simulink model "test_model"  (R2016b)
settings: Solver=VariableStepAuto  StartTime=0.0  StopTime=runtime  RelTol=1e-3
InitFcn:
  | clear mex
  | delete test_model_sfun.mexw64
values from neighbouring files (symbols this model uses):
  g = 9.81    [modelParameters.m]
  height_controlled_o = (((Rm*If        + (((omega0_o * 2 * Rm * Kv * Kq      * Kd + 1)^2) - 1)/(4* Rm*Kv^2*Kq      * Kd))/Vb)*(Pmax - Pmin) + Pmin)    [modelParameters.m]
  If = 0.3836    [modelParameters.m]
  Jreq = 4.2012e-05    [modelParameters.m]
  Jxx = 0.0130    (= 0.013)    [modelParameters.m]
  Jyy = 0.0140    (= 0.014)    [modelParameters.m]
  Jzz = 0.0285    [modelParameters.m]
  Kd = 1.4852e-07    [modelParameters.m]
  Ki_mahony = 0.001    [modelParameters.m]
  Kp_mahony = 0.4    [modelParameters.m]
  Kq = 96.3422    [modelParameters.m]
  Kt = 1.2007e-05    [modelParameters.m]
  Kv = 96.3422    [modelParameters.m]
  m = 1.216    [modelParameters.m]
  omega0_o = sqrt((m*g)/(4*Kt))    [modelParameters.m]
  omega1_o = sqrt((m*g)/(4*Kt))    [modelParameters.m]
  omega2_o = sqrt((m*g)/(4*Kt))    [modelParameters.m]
  omega3_o = sqrt((m*g)/(4*Kt))    [modelParameters.m]
  pitch_o = 0    [modelParameters.m]
  pitchrate_o = 0    [modelParameters.m]
  Pmax = 1    [modelParameters.m]
  Pmin = 0    [modelParameters.m]
  r_oc = [0; 0; 0]    [modelParameters.m]
  rhx = 0.16    [modelParameters.m]
  rhy = 0.16    [modelParameters.m]
  rhz = 0.03    [modelParameters.m]
  Rm = 0.235    [modelParameters.m]
  roll_o = 0    [modelParameters.m]
  rollrate_o = 0    [modelParameters.m]
  Tc = 0.04    [modelParameters.m]
  Tq = 0.005    [modelParameters.m]
  Vb = 11.4    [modelParameters.m]
  x_controlled_o = 0    [modelParameters.m]
  x_o = 0    [modelParameters.m]
  x_vel_o = 0    [modelParameters.m]
  y_controlled_o = 0    [modelParameters.m]
  y_o = 0    [modelParameters.m]
  y_vel_o = 0    [modelParameters.m]
  yaw_controlled_o = 0    [modelParameters.m]
  yaw_o = 0    [modelParameters.m]
  yawrate_o = 0    [modelParameters.m]
  z_o = 0    [modelParameters.m]
  z_vel_o = 0    [modelParameters.m]
undefined symbols (not defined in the file or in its folder): a, Ki, Kp, Ts
libraries: simulink x38, dsparch4 x3, vrlib x2
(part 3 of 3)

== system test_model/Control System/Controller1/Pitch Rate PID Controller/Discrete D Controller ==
  pitch_angle : Inport
  Discrete Derivative : simulink/Discrete/Discrete Derivative  gainval=Kd  ICPrevScaledInput=0.0  OutMin=[]  OutMax=[]  OutDataType=fixdt(1, 16)  OutScaling=2^-10  DoSatur=off
  Discrete Filter : DiscreteFilter  Numerator=[0 a]  Denominator=[1-a]
  Sum : Sum  Inputs=|++
  output : Outport
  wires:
  Discrete Derivative/1 -> Sum/1
  Discrete Filter/1 -> Sum/2
  Sum/1 -> Discrete Filter/1, output/1
  pitch_angle/1 -> Discrete Derivative/1

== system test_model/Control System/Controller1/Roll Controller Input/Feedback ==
  roll_error_model : Inport
  roll_error : Outport
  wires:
  roll_error_model/1 -> roll_error/1

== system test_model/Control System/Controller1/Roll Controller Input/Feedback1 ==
  roll_angle_model : Inport
  roll_angle : Outport
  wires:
  roll_angle_model/1 -> roll_angle/1

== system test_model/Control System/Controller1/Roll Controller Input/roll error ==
  From Workspace1 : FromWorkspace  VariableName=roll_angle  SampleTime=Tq  Interpolate=off  OutputAfterFinalValue=Holding final value
  From Workspace4 : FromWorkspace  VariableName=roll_error  SampleTime=Tq  Interpolate=off  OutputAfterFinalValue=Holding final value
  roll_error : Outport
  roll_angle : Outport  Port=2
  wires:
  From Workspace4/1 -> roll_error/1
  From Workspace1/1 -> roll_angle/1

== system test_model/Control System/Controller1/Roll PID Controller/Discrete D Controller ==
  pitch_angle : Inport
  Discrete Derivative : simulink/Discrete/Discrete Derivative  gainval=Kd  ICPrevScaledInput=0.0  OutMin=[]  OutMax=[]  OutDataType=fixdt(1, 16)  OutScaling=2^-10  DoSatur=off
  Discrete Filter : DiscreteFilter  Numerator=[0 a]  Denominator=[1-a]
  Sum : Sum  Inputs=|++
  output : Outport
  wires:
  Discrete Derivative/1 -> Sum/1
  Discrete Filter/1 -> Sum/2
  Sum/1 -> Discrete Filter/1, output/1
  pitch_angle/1 -> Discrete Derivative/1

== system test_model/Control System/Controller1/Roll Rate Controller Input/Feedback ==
  rollrate_error_model : Inport
  rollrate_error : Outport
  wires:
  rollrate_error_model/1 -> rollrate_error/1

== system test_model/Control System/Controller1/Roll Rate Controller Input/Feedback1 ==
  rollrate_model : Inport
  rollrate : Outport
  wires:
  rollrate_model/1 -> rollrate/1

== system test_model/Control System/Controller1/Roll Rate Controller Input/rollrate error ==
  From Workspace1 : FromWorkspace  VariableName=rollrate  SampleTime=Tq  Interpolate=off  OutputAfterFinalValue=Holding final value
  From Workspace5 : FromWorkspace  VariableName=rollrate_error  SampleTime=Tq  Interpolate=off  OutputAfterFinalValue=Holding final value
  rollrate_error : Outport
  rollrate : Outport  Port=2
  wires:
  From Workspace5/1 -> rollrate_error/1
  From Workspace1/1 -> rollrate/1

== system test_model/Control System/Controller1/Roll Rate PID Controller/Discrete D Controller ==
  pitch_angle : Inport
  Discrete Derivative : simulink/Discrete/Discrete Derivative  gainval=Kd  ICPrevScaledInput=0.0  OutMin=[]  OutMax=[]  OutDataType=fixdt(1, 16)  OutScaling=2^-10  DoSatur=off
  Discrete Filter : DiscreteFilter  Numerator=[0 a]  Denominator=[1-a]
  Sum : Sum  Inputs=|++
  output : Outport
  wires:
  Discrete Derivative/1 -> Sum/1
  Discrete Filter/1 -> Sum/2
  Sum/1 -> Discrete Filter/1, output/1
  pitch_angle/1 -> Discrete Derivative/1

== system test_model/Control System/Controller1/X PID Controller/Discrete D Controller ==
  x_pos : Inport
  Discrete Derivative : simulink/Discrete/Discrete Derivative  gainval=Kd  ICPrevScaledInput=0.0  OutMin=[]  OutMax=[]  OutDataType=fixdt(1, 16)  OutScaling=2^-10  DoSatur=off
  Discrete Filter : DiscreteFilter  Numerator=[0 a]  Denominator=[1-a]
  Sum : Sum  Inputs=|++
  output : Outport
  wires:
  Discrete Derivative/1 -> Sum/1
  Discrete Filter/1 -> Sum/2
  Sum/1 -> Discrete Filter/1, output/1
  x_pos/1 -> Discrete Derivative/1

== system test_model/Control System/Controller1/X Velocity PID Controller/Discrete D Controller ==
  x_vel : Inport
  Discrete Derivative : simulink/Discrete/Discrete Derivative  gainval=1.0  ICPrevScaledInput=0.0  OutMin=[]  OutMax=[]  OutDataType=fixdt(1, 16)  OutScaling=2^-10  DoSatur=off
  Discrete Filter : DiscreteFilter  Numerator=[0 a]  Denominator=[1-a]
  Sum : Sum  Inputs=|++
  output : Outport
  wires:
  Discrete Derivative/1 -> Sum/1
  Discrete Filter/1 -> Sum/2
  Sum/1 -> Discrete Filter/1, output/1
  x_vel/1 -> Discrete Derivative/1

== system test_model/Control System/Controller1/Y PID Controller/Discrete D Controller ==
  y_pos : Inport
  Discrete Derivative : simulink/Discrete/Discrete Derivative  gainval=1.0  ICPrevScaledInput=0.0  OutMin=[]  OutMax=[]  OutDataType=fixdt(1, 16)  OutScaling=2^-10  DoSatur=off
  Discrete Filter : DiscreteFilter  Numerator=[0 a]  Denominator=[1-a]
  Sum : Sum  Inputs=|++
  output : Outport
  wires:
  Discrete Derivative/1 -> Sum/1
  Discrete Filter/1 -> Sum/2
  Sum/1 -> Discrete Filter/1, output/1
  y_pos/1 -> Discrete Derivative/1

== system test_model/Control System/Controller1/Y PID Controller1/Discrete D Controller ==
  y_pos : Inport
  Discrete Derivative : simulink/Discrete/Discrete Derivative  gainval=1.0  ICPrevScaledInput=0.0  OutMin=[]  OutMax=[]  OutDataType=fixdt(1, 16)  OutScaling=2^-10  DoSatur=off
  Discrete Filter : DiscreteFilter  Numerator=[0 a]  Denominator=[1-a]
  Sum : Sum  Inputs=|++
  output : Outport
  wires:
  Discrete Derivative/1 -> Sum/1
  Discrete Filter/1 -> Sum/2
  Sum/1 -> Discrete Filter/1, output/1
  y_pos/1 -> Discrete Derivative/1

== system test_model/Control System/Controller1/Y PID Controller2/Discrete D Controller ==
  x_pos : Inport
  Discrete Derivative : simulink/Discrete/Discrete Derivative  gainval=1.0  ICPrevScaledInput=0.0  OutMin=[]  OutMax=[]  OutDataType=fixdt(1, 16)  OutScaling=2^-10  DoSatur=off
  Discrete Filter : DiscreteFilter  Numerator=[0 a]  Denominator=[1-a]
  Sum : Sum  Inputs=|++
  output : Outport
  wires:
  Discrete Derivative/1 -> Sum/1
  Discrete Filter/1 -> Sum/2
  Sum/1 -> Discrete Filter/1, output/1
  x_pos/1 -> Discrete Derivative/1

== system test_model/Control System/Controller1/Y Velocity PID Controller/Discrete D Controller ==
  y_pos : Inport
  Discrete Derivative : simulink/Discrete/Discrete Derivative  gainval=1.0  ICPrevScaledInput=0.0  OutMin=[]  OutMax=[]  OutDataType=fixdt(1, 16)  OutScaling=2^-10  DoSatur=off
  Discrete Filter : DiscreteFilter  Numerator=[0 a]  Denominator=[1-a]
  Sum : Sum  Inputs=|++
  output : Outport
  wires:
  Discrete Derivative/1 -> Sum/1
  Discrete Filter/1 -> Sum/2
  Sum/1 -> Discrete Filter/1, output/1
  y_pos/1 -> Discrete Derivative/1

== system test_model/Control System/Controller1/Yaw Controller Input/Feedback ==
  yaw_error_model : Inport
  yaw_error : Outport
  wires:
  yaw_error_model/1 -> yaw_error/1

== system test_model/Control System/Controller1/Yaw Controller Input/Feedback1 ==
  yaw_angle_model : Inport
  yaw_angle : Outport
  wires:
  yaw_angle_model/1 -> yaw_angle/1

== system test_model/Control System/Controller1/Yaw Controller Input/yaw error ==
  From Workspace1 : FromWorkspace  VariableName=yaw_angle  SampleTime=Tc  Interpolate=off  OutputAfterFinalValue=Holding final value
  From Workspace7 : FromWorkspace  VariableName=yaw_error  SampleTime=Tc  Interpolate=off  OutputAfterFinalValue=Holding final value
  yaw_error : Outport
  yaw_angle : Outport  Port=2
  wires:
  From Workspace7/1 -> yaw_error/1
  From Workspace1/1 -> yaw_angle/1

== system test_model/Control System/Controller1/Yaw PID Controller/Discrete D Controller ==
  yaw_pos : Inport
  Discrete Derivative : simulink/Discrete/Discrete Derivative  gainval=1.0  ICPrevScaledInput=0.0  OutMin=[]  OutMax=[]  OutDataType=fixdt(1, 16)  OutScaling=2^-10  DoSatur=off
  Discrete Filter : DiscreteFilter  Numerator=[0 a]  Denominator=[1-a]
  Sum : Sum  Inputs=|++
  output : Outport
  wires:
  Discrete Derivative/1 -> Sum/1
  Discrete Filter/1 -> Sum/2
  Sum/1 -> Discrete Filter/1, output/1
  yaw_pos/1 -> Discrete Derivative/1

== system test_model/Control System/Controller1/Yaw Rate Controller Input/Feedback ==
  yawrate_error_model : Inport
  yawrate_error : Outport
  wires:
  yawrate_error_model/1 -> yawrate_error/1

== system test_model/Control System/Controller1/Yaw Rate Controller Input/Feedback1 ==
  yawrate_model : Inport
  yawrate : Outport
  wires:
  yawrate_model/1 -> yawrate/1

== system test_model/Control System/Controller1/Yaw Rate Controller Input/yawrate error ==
  From Workspace1 : FromWorkspace  VariableName=yawrate  SampleTime=Tq  Interpolate=off  OutputAfterFinalValue=Holding final value
  From Workspace8 : FromWorkspace  VariableName=yawrate_error  SampleTime=Tq  Interpolate=off  OutputAfterFinalValue=Holding final value
  yawrate_error : Outport
  yawrate : Outport  Port=2
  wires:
  From Workspace8/1 -> yawrate_error/1
  From Workspace1/1 -> yawrate/1

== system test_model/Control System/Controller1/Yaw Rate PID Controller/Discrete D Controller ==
  yawrate : Inport
  Discrete Derivative : simulink/Discrete/Discrete Derivative  gainval=Kd  ICPrevScaledInput=0.0  OutMin=[]  OutMax=[]  OutDataType=fixdt(1, 16)  OutScaling=2^-10  DoSatur=off
  Discrete Filter : DiscreteFilter  Numerator=[0 a]  Denominator=[1-a]
  Sum : Sum  Inputs=|++
  output : Outport
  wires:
  Discrete Derivative/1 -> Sum/1
  Discrete Filter/1 -> Sum/2
  Sum/1 -> Discrete Filter/1, output/1
  yawrate/1 -> Discrete Derivative/1

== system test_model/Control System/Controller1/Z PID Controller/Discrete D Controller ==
  z_pos : Inport
  Discrete Derivative : simulink/Discrete/Discrete Derivative  gainval=1.0  ICPrevScaledInput=0.0  OutMin=[]  OutMax=[]  OutDataType=fixdt(1, 16)  OutScaling=2^-10  DoSatur=off
  Discrete Filter : DiscreteFilter  Numerator=[0 a]  Denominator=[1-a]
  Sum : Sum  Inputs=|++
  output : Outport
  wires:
  Discrete Derivative/1 -> Sum/1
  Discrete Filter/1 -> Sum/2
  Sum/1 -> Discrete Filter/1, output/1
  z_pos/1 -> Discrete Derivative/1

== matlab function test_model/Actuation/Gravity

 ==
function E_Fg = gravity(m, g)

E_Fg = [0; 0; m*g];

== matlab function test_model/Actuation/Lbe





 ==
function E_ro  = linear_body_earth_conversion(B_vo, euler_angles)

euler_rates = zeros(3,1);
E_ro = zeros(3,1);

phi = euler_angles(1);
theta = euler_angles(2);
psi = euler_angles(3);

Leb = [cos(theta)*cos(psi), sin(phi)*sin(theta)*cos(psi)-cos(phi)*sin(psi), cos(phi)*sin(theta)*cos(psi)+sin(phi)*sin(psi); ...
       cos(theta)*sin(psi), sin(phi)*sin(theta)*sin(psi)+cos(phi)*cos(psi), cos(phi)*sin(theta)*sin(psi)-sin(phi)*cos(psi); ...
           -sin(theta)    ,                sin(phi)*cos(theta)            ,                 cos(phi)*cos(theta)           ];

E_ro = Leb * B_vo;

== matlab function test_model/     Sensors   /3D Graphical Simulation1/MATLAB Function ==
function y = eigenaxis_ucart(u)


if abs(u(1))< 0.0001
    u(1) = 0.0001;
end

if abs(u(2))< 0.0001
    u(2) = 0.0001;
end

if abs(u(3))< 0.0001
    u(3) = 0.0001;
end

u = [ -u(1); -u(2); u(3) ];% [Pitch, Yaw, Roll] 

C11 = cos(u(2))*cos(u(3));
C12 = cos(u(2))*sin(u(3));
C13 = -sin(u(2));
C21 = sin(u(1))*sin(u(2))*cos(u(3))-cos(u(1))*sin(u(3));
C22 = sin(u(1))*sin(u(2))*sin(u(3))+cos(u(1))*cos(u(3));
C23 = sin(u(1))*cos(u(2));
C31 = cos(u(1))*sin(u(2))*cos(u(3))+sin(u(1))*sin(u(3));
C32 = cos(u(1))*sin(u(2))*sin(u(3))-sin(u(1))*cos(u(3));
C33 = cos(u(1))*cos(u(2));
    
theta = acos(0.5*(C11+C22+C33-1));

e = [C23-C32; C31-C13; C12-C21]/(2*sin(theta));
    
y = [e; theta];

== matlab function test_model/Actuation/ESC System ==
function Vb_eff   = ESC(P, Pmin, Pmax, Vb)

P1 = P(1);
P2 = P(2);
P3 = P(3);
P4 = P(4);

% Define u_Pi for each of the rotors, limiting it to be greater than 0
% u_P0 = (rotor_0_duty_cycle/100 - Pmin) / (Pmax - Pmin);
% u_P1 = (rotor_1_duty_cycle/100 - Pmin) / (Pmax - Pmin);
% u_P2 = (rotor_2_duty_cycle/100 - Pmin) / (Pmax - Pmin);
% u_P3 = (rotor_3_duty_cycle/100 - Pmin) / (Pmax - Pmin);
u_P0 = (P1 - Pmin) / (Pmax - Pmin);
u_P1 = (P2 - Pmin) / (Pmax - Pmin);
u_P2 = (P3 - Pmin) / (Pmax - Pmin);
u_P3 = (P4 - Pmin) / (Pmax - Pmin);


% Determine the effective battery voltage from each ESC
Vb_eff_0 = u_P0 * Vb;
Vb_eff_1 = u_P1 * Vb;
Vb_eff_2 = u_P2 * Vb;
Vb_eff_3 = u_P3 * Vb;
    
Vb_eff = [Vb_eff_0, Vb_eff_1, Vb_eff_2, Vb_eff_3];

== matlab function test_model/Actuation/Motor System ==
function w_dot = motor(Vb_eff, w, Rm, Kv, Kq, Kd, If, Jreq)

% Define each motors effective battery voltage
Vb_eff_0 = Vb_eff(1);
Vb_eff_1 = Vb_eff(2);
Vb_eff_2 = Vb_eff(3);
Vb_eff_3 = Vb_eff(4);

% Determine the angular velocity of each rotor from feedback
w_0 = w(1);
w_1 = w(2);
w_2 = w(3);
w_3 = w(4);

% Determine angular acceleration of each rotor
w_0_dot = 1/(Jreq*Rm*Kq) * Vb_eff_0 - 1/(Jreq*Rm*Kq*Kv) * w_0 - 1/(Jreq*Kq)*If - (Kd/Jreq) * w_0^2;
w_1_dot = 1/(Jreq*Rm*Kq) * Vb_eff_1 - 1/(Jreq*Rm*Kq*Kv) * w_1 - 1/(Jreq*Kq)*If - (Kd/Jreq) * w_1^2;
w_2_dot = 1/(Jreq*Rm*Kq) * Vb_eff_2 - 1/(Jreq*Rm*Kq*Kv) * w_2 - 1/(Jreq*Kq)*If - (Kd/Jreq) * w_2^2;
w_3_dot = 1/(Jreq*Rm*Kq) * Vb_eff_3 - 1/(Jreq*Rm*Kq*Kv) * w_3 - 1/(Jreq*Kq)*If - (Kd/Jreq) * w_3^2;

w_dot = [w_0_dot, w_1_dot, w_2_dot, w_3_dot];

== matlab function test_model/Actuation/Rotor System







 ==
function [B_omega_dot, B_vo_dot]= rotor(w_dot, w, B_Fg, B_omega, B_vo, m, Kt, Kd, rhx, rhy, rhz, Jreq, Jxx, Jyy, Jzz, r_oc)

% Create J vector
J = [Jxx,  0 ,  0 ; ...
      0 , Jyy,  0 ; ...
      0 ,  0 , Jzz;];
  
r_oc_X = [0, -r_oc(3), r_oc(2); r_oc(3), 0, -r_oc(1); -r_oc(2), r_oc(1), 0];

% Create r_hi vector
rh_0 = [-rhx; rhy; -rhz];
rh_1 = [rhx; rhy; -rhz];
rh_2 = [-rhx; -rhy; -rhz];
rh_3 = [rhx; -rhy; -rhz];

% Define 3x3 Identity Matrix
I = eye(3);

% Create gamma vectors
gamma_Ti = [0; 0; -1];
gamma_omega_03 = [0; 0; 1];  %Rotors 0 and 3 use this gamma_omega vector
gamma_omega_12 = [0; 0; -1]; %Rotors 1 and 2 use this gamma_omega vector

% Define angular velocities for each rotor
w_0 = w(1);
w_1 = w(2);
w_2 = w(3);
w_3 = w(4);

% Define angular acceleration for each rotor
w_0_dot = w_dot(1);
w_1_dot = w_dot(2);
w_2_dot = w_dot(3);
w_3_dot = w_dot(4);

% Define the rotor force in the z-direction from each rotor
B_Fr_0 = Kt * w_0 * w_0 * gamma_Ti;
B_Fr_1 = Kt * w_1 * w_1 * gamma_Ti;
B_Fr_2 = Kt * w_2 * w_2 * gamma_Ti;
B_Fr_3 = Kt * w_3 * w_3 * gamma_Ti;

% Sum up the rotor forces in the z-direction from each vector to get the
% total body force in the z-direction
B_Fr = B_Fr_0 + B_Fr_1 + B_Fr_2 + B_Fr_3;

% Define the in-plane drag and induced torque produced by each rotor
 B_Q_d0 = -1 * Kd * w_0 * w_0 * gamma_omega_03;
 B_Q_d1 = -1 * Kd * w_1 * w_1 * gamma_omega_12;
 B_Q_d2 = -1 * Kd * w_2 * w_2 * gamma_omega_12;
 B_Q_d3 = -1 * Kd * w_3 * w_3 * gamma_omega_03;

% Sum up the total in-plane drag and induced torque to get the total
% in-plane drag and induced torque on the body
B_Q_d = B_Q_d0 + B_Q_d1 + B_Q_d2 + B_Q_d3;

% Define the force lever arm torque created from the force produced by each
% rotor in the z-direction
B_Q_F0 = cross( rh_0, B_Fr_0 );
B_Q_F1 = cross( rh_1, B_Fr_1 );
B_Q_F2 = cross( rh_2, B_Fr_2 );
B_Q_F3 = cross( rh_3, B_Fr_3 );

B_Q_F = B_Q_F0 + B_Q_F1 + B_Q_F2 + B_Q_F3;

%Define the change in angular momentum torque produced by each rotor 
B_Q_L0 = -1 * Jreq * ( cross(B_omega, w_0 * gamma_omega_03) + w_0_dot * gamma_omega_03 );
B_Q_L1 = -1 * Jreq * ( cross(B_omega, w_1 * gamma_omega_12) + w_1_dot * gamma_omega_12 ); 
B_Q_L2 = -1 * Jreq * ( cross(B_omega, w_2 * gamma_omega_12) + w_2_dot * gamma_omega_12 ); 
B_Q_L3 = -1 * Jreq * ( cross(B_omega, w_3 * gamma_omega_03) + w_3_dot * gamma_omega_03 );

% Sum up the total change in angular momentum torque produced by each rotor
B_Q_L = B_Q_L0 + B_Q_L1 + B_Q_L2 + B_Q_L3;

% Define the total rotor system torque as the sum of the in-plane drag and
% induced torque, force lever arm torque, and change in angular momentum
% torques
B_Q = B_Q_d + B_Q_F + B_Q_L;

% Define the body forces in the z-direction from each vector to get the
% total body force in the z-direction
B_F = B_Fr + B_Fg; 

% Determine the dynamics of the system
M = [m * I , -m * r_oc_X; 
    zeros(3,3), J];

dynamics = M^(-1) *     [B_F - cross( B_omega, m*(B_vo + cross(B_omega, r_oc))); ...
     B_Q - cross(B_omega, J * B_omega) - cross(r_oc, B_F)];

% Define the body frame angular velocities
B_vo_dot = dynamics(1:3);

% Define the body frame linear velocities
B_omega_dot = dynamics(4:6);
 
% B_vo_dot = (m*I)^(-1) * ( B_F - cross( B_omega, m*(B_vo + cross(B_omega, r_oc)) ) );
% B_omega_dot = J ^(-1) * ( B_Q - cross(B_omega, J * B_omega) - cross(r_oc, B_F)  );

== matlab function test_model/Actuation/Aeb














 ==
function euler_rates = angular_body_earth_conversion(B_omega, euler_angles)

phi = euler_angles(1);
theta = euler_angles(2);

Aeb = [1,  sin(phi)*tan(theta), cos(phi)*tan(theta); ...
       0,      cos(phi)       ,        -sin(phi)   ; ...
       0,  sin(phi)/cos(theta), cos(phi)/cos(theta)];

   
euler_rates = Aeb * B_omega;

== matlab function test_model/Actuation/Lbe

















 ==
function [B_Fg, B_g]  = linear_earth_body_conversion(E_Fg, euler_angles, m)

phi = euler_angles(1);
theta = euler_angles(2);
psi = euler_angles(3);

Lbe = [             cos(theta)*cos(psi)              ,          cos(theta)*sin(psi)                  ,     -sin(theta)    ; ...
       sin(phi)*sin(theta)*cos(psi)-cos(phi)*sin(psi), sin(phi)*sin(theta)*sin(psi)+cos(phi)*cos(psi), sin(phi)*cos(theta); ...
       cos(phi)*sin(theta)*cos(psi)+sin(phi)*sin(psi), cos(phi)*sin(theta)*sin(psi)-sin(phi)*cos(psi), cos(phi)*cos(theta)];

B_Fg = Lbe * E_Fg;

B_g = B_Fg/m;

== matlab function test_model/     Sensors   /IMU





/






 ==
function [accelReading,gyroReading] = idealIMU(B_vo_dot, B_vo, B_Omega, B_g, g, r_oc)
%#codegen

a = B_vo_dot + cross(B_Omega,B_vo); % body frame acceleration 

accelReading = (a - B_g)/g ; % accelerometer reading (ideal)

gyroReading = B_Omega ; % gyroscope reading (ideal) 

end

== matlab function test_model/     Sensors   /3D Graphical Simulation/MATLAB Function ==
function y = eigenaxis_ucart(u)


if abs(u(1))< 0.0001
    u(1) = 0.0001;
end

if abs(u(2))< 0.0001
    u(2) = 0.0001;
end

if abs(u(3))< 0.0001
    u(3) = 0.0001;
end

u = [ -u(1); -u(2); u(3) ];% [Pitch, Yaw, Roll] 

C11 = cos(u(2))*cos(u(3));
C12 = cos(u(2))*sin(u(3));
C13 = -sin(u(2));
C21 = sin(u(1))*sin(u(2))*cos(u(3))-cos(u(1))*sin(u(3));
C22 = sin(u(1))*sin(u(2))*sin(u(3))+cos(u(1))*cos(u(3));
C23 = sin(u(1))*cos(u(2));
C31 = cos(u(1))*sin(u(2))*cos(u(3))+sin(u(1))*sin(u(3));
C32 = cos(u(1))*sin(u(2))*sin(u(3))-sin(u(1))*cos(u(3));
C33 = cos(u(1))*cos(u(2));
    
theta = acos(0.5*(C11+C22+C33-1));

e = [C23-C32; C31-C13; C12-C21]/(2*sin(theta));
    
y = [e; theta];

== matlab function test_model/     Sensors   /Aeb









 ==
function euler_rates_IMU = angular_body_earth_conversion(gyro_reading, euler_angles_filtered)

phi = euler_angles_filtered(1);
theta = euler_angles_filtered(2);

Aeb = [1, sin(phi)*tan(theta), cos(phi)*tan(theta); ...
       0,     cos(phi)       ,        -sin(phi)   ; ...
       0,  sin(phi)/cos(theta), cos(phi)/cos(theta)];

   
euler_rates_IMU = Aeb * gyro_reading;

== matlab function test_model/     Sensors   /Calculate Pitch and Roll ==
function [accel_pitch, accel_roll] = getPitchAndRoll(accel_reading)

x_accel = accel_reading(1);
y_accel = accel_reading(2);
z_accel = accel_reading(3);

accel_pitch = atan(x_accel/sqrt(y_accel^2 + z_accel^2));
accel_roll = atan( -y_accel/( sqrt(z_accel^2 + x_accel^2))  );

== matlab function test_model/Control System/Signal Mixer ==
function P  = signal_mixer(height_controlled, y_controlled, x_controlled, yaw_controlled)

controller_outputs = [ height_controlled; x_controlled; y_controlled; yaw_controlled ];
signal_mixer = [ 1, -1, -1, -1; ... 
                 1,  1, -1,  1; ...
                 1, -1,  1,  1; ...
                 1,  1,  1, -1 ];

% signal_mixer = [ 1,  1, -1, -1; ... 
%                  1, -1, -1,  1; ...
%                  1,  1,  1,  1; ...
%                  1, -1,  1, -1 ];
             
P = signal_mixer * controller_outputs;

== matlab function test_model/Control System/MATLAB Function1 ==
function [z_corr, y_cor, x_corr, yaw_corr, pid_y_out, pid_roll_out] = c_controller(set_x, set_y, set_z, set_yaw, ...
    cur_x, cur_y, cur_z, ...
    cur_phi, cur_theta, cur_psi, ...
    cur_phi_d, cur_theta_d, cur_psi_d, vrpn_id, Tc)

out_z = -1;
out_y = -1;
out_x = -1;
out_yaw = -1;
c_pid_y = -1;
c_pid_roll = -1;

coder.ceval('c_controller', vrpn_id, Tc, set_x, set_y, set_z, set_yaw, ...
                    cur_x, cur_y, cur_z, ...
                    cur_phi, cur_theta, cur_psi, ...
                    cur_phi_d, cur_theta_d, cur_psi_d, ...
                    coder.wref(out_z), coder.wref(out_y), coder.wref(out_x), coder.wref(out_yaw), ...
                    coder.wref(c_pid_y), coder.wref(c_pid_roll));

z_corr = out_z;
y_cor = out_y;
x_corr = out_x;
pid_y_out = c_pid_y;
pid_roll_out = c_pid_roll;
yaw_corr = out_yaw;

== matlab function test_model/     Sensors   /Aeb_c









1 ==
function euler_rates_IMU = angular_body_earth_conversion(gyro_reading, euler_angles_filtered)

phi = euler_angles_filtered(1);
theta = euler_angles_filtered(2);
psi = NaN;

phi_dot = -1;
theta_dot = -1;
psi_dot = -1;

p = gyro_reading(1);
q = gyro_reading(2);
r = gyro_reading(3);

coder.ceval( 'aeb_mat', p, q, r, phi, theta, psi, coder.wref(phi_dot), ...
    coder.wref(theta_dot), coder.wref(psi_dot) );

   
euler_rates_IMU = [phi_dot; theta_dot; psi_dot];

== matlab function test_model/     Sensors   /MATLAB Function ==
function euler_angles_IMU  = complimentaryFilterC(accel_pitch, accel_roll, euler_rates_gyro)

euler_x = euler_rates_gyro(1);
euler_y = euler_rates_gyro(2);

filtered_pitch = -1;
filtered_roll = -1;

coder.ceval('compl_filter', accel_pitch, accel_roll, euler_x, euler_y, ...
            coder.wref(filtered_pitch), coder.wref(filtered_roll));

euler_angles_IMU = [filtered_roll; filtered_pitch];

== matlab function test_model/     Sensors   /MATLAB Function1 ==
function [accel_pitch, accel_roll]  = angle_IMU_C(accel_reading)

accel_x = accel_reading(1);
accel_y = accel_reading(2);
accel_z = accel_reading(3);

calculated_pitch = -1;
calculated_roll = -1;

coder.ceval('angle_accel', accel_x, accel_y, accel_z, coder.wref(calculated_pitch), coder.wref(calculated_roll));

accel_pitch = calculated_pitch;
accel_roll = calculated_roll;

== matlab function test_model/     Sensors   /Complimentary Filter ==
function euler_angles_IMU   = complimentaryFilter(accel_pitch, accel_roll, euler_rates_gyro, prev_euler_angles)

k_gyro = 0.99; 
k_accel = 1-k_gyro; 

Ts = 0.005; % 5 milliseconds

prev_phi = prev_euler_angles(1);
prev_theta = prev_euler_angles(2);

prev_phi_dot = euler_rates_gyro(1);
prev_theta_dot = euler_rates_gyro(2);

integrated_phi_gyro = Ts * prev_phi_dot + prev_phi;
integrated_theta_gyro = Ts * prev_theta_dot + prev_theta;

phi = k_gyro * integrated_phi_gyro + k_accel * accel_roll;
theta = k_gyro * integrated_theta_gyro + k_accel * accel_pitch;

euler_angles_IMU = [phi; theta];

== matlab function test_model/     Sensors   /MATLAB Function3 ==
function [eulerAngles, integralFeedback, quaternions] = ...
    mahonyFilter(accelReadings, gyroReadings, quaternions_prev, ...
    integralFeedback_prev, Tq, Kp_mahony, Ki_mahony)
%     mahonyFilter(accelReadings, gyroReadings, eulerAngles_prev, ...
%     integralFeedback_prev, Tq, Kp_mahony, Ki_mahony)
    
    
    %Save quadcopter loop time as dt
    dt = Tq;

    %Pull accelerometer readings and negate them to compare
    accel_x = accelReadings(1);
    accel_y = accelReadings(2);
    accel_z = accelReadings(3);
    
    %Negate the accelerometer values to compare with direction of the
    %gravity vector
    accel_x = (-1) * accel_x;
    accel_y = (-1) * accel_y;
    accel_z = (-1) * accel_z;

    %Pull gyroscope readings
    gyro_x = gyroReadings(1);
    gyro_y = gyroReadings(2);
    gyro_z = gyroReadings(3);

    %Pull previous Euler angles
%     roll_prev = eulerAngles_prev(1);
%     pitch_prev = eulerAngles_prev(2);
%     yaw_prev = eulerAngles_prev(3);
    
    %Pull previous integral feedback terms
    integralFeedback_x_prev = integralFeedback_prev(1);
    integralFeedback_y_prev = integralFeedback_prev(2);
    integralFeedback_z_prev = integralFeedback_prev(3);

    %Calculate half cosines and sines for the quaternion elements
%     cosHalfRoll = cos( 0.5 * roll_prev );
%     sinHalfRoll = sin( 0.5 * roll_prev );
%     cosHalfPitch = cos( 0.5 * pitch_prev );
%     sinHalfPitch = sin( 0.5 * pitch_prev );
%     cosHalfYaw = cos( 0.5 * yaw_prev );
%     sinHalfYaw = sin( 0.5 * yaw_prev );

    %Calculate the quaternion elements
%     q0 = cosHalfRoll * cosHalfPitch * cosHalfYaw + ...
%         sinHalfRoll * sinHalfPitch * sinHalfYaw;
% 
%     q1 = sinHalfRoll * cosHalfPitch * cosHalfYaw - ...
%         cosHalfRoll * sinHalfPitch * sinHalfYaw;
% 
%     q2 = cosHalfRoll * sinHalfPitch * cosHalfYaw + ...
%         sinHalfRoll * cosHalfPitch * sinHalfYaw;
% 
%     q3 = (-1) * sinHalfRoll * sinHalfPitch * cosHalfYaw + ...
%         cosHalfRoll * cosHalfPitch * sinHalfYaw;

    %Pull the quaternion values
    q0 = quaternions_prev(1);
    q1 = quaternions_prev(2);
    q2 = quaternions_prev(3);
    q3 = quaternions_prev(4);


    %Calculate the rate of change of the quaternion from the gyroscope
%     q0_dot = 0.5 * ( (-1)*(q1 * gyro_x) - (q2 * gyro_y) - (q3 * gyro_z) );
%     q1_dot = 0.5 * ( (q0 * gyro_x) + (q2 * gryo_z) - (q3 * gyro_y) );
%     q2_dot = 0.5 * ( (q0 * gyro_y) - (q1 * gyro_z) + (q3 * gyro_x) );
%     q3_dot = 0.5 * ( (q0 * gyro_z) + (q1 * gyro_y) - (q2 * gyro_x) );

    %Define initial values for the corrected gyroscope values
    gyro_x_corrected = gyro_x;
    gyro_y_corrected = gyro_y;
    gyro_z_corrected = gyro_z;
    
    %Define initial values for the corrected integral feedback values
    integralFeedback_x = integralFeedback_x_prev;
    integralFeedback_y = integralFeedback_y_prev;
    integralFeedback_z = integralFeedback_z_prev;

    %Only compute the feedback if the accelerometer measurements are valid
    %This prevents NaN values when normalizing the accelerometer measurements
    if( accel_x ~= 0 && accel_y ~= 0  && accel_z ~= 0 )

       %Check... maybe we don't need to do this normalization...
       %Ideally our accelerometer readings should have a magnitude of 1, but
       %this is usually not the case with data we have collected
       accel_mag = ( (accel_x ^ 2) + (accel_y ^ 2) + (accel_z ^ 2) ) ^ 0.5;
       accel_x = accel_x / accel_mag;
       accel_y = accel_y / accel_mag;
       accel_z = accel_z / accel_mag;

       %Estimate direction of gravity
       vx = 2 * ( (q1 * q3) - (q0 * q2) );
       vy = 2 * ( (q0 * q1) + (q2 * q3) );
       vz = (2 * q0 * q0) - (q3 * q3);
       
       %Error is the sum of the cross product between the estimated and
       %measured direction of gravity
       ex = (accel_y * vz) - (accel_z * vy);
       ey = (accel_z * vx) - (accel_x * vz);
       ez = (accel_x * vy) - (accel_y * vx);
       
       %Compute and apply the proportional feedback
       gyro_x_corrected = gyro_x + (Kp_mahony * ex);
       gyro_y_corrected = gyro_y + (Kp_mahony * ey);
       gyro_z_corrected = gyro_z + (Kp_mahony * ez);

       %Compute and apply the integral feedback, if it is enabled
       if ( Ki_mahony > 0 )
           
           %Integrate digitally based on sample time and scale by Ki, and
           %accumulate the integral term by adding this to the previous
           %feedback term
           integralFeedback_x = (Ki_mahony * ex * dt) + ...
               integralFeedback_x_prev;
           integralFeedback_y = (Ki_mahony * ey * dt) + ...
               integralFeedback_y_prev;
           integralFeedback_z = (Ki_mahony * ez * dt) + ...
               integralFeedback_z_prev;
           
           %Correct the gyroscope values using the new integral feedback
           gyro_x_corrected = gyro_x_corrected + integralFeedback_x;
           gyro_y_corrected = gyro_y_corrected + integralFeedback_y;
           gyro_z_corrected = gyro_z_corrected + integralFeedback_z;
           
       else
           
           %Otherwise, reset the integral terms to zero to prevent windup
           integralFeedback_x = 0;
           integralFeedback_y = 0;
           integralFeedback_z = 0;
           
       end %if ( Ki_mahoney > 0 )

    end %if ( accel_x ~= 0 && accel_y ~= 0 && accel_z ~= 0 )

    %Integrate the rate of change of the quaternion
    %First, pre-multiply the common factors to the gyro reading values
    gyro_x_corrected = gyro_x_corrected * (0.5 * dt);
    gyro_y_corrected = gyro_y_corrected * (0.5 * dt);
    gyro_z_corrected = gyro_z_corrected * (0.5 * dt);
    
    %Now, create temporary variales for the first three quaternion values
    qa = q0;
    qb = q1;
    qc = q2;
    
    %Now perform calculation to integrate the rate of the quaternion
    q0 = q0 - (qb * gyro_x_corrected) - (qc * gyro_y_corrected) - ...
        (q3 * gyro_z_corrected);
    q1 = q1 + (qa * gyro_x_corrected) + (qc * gyro_z_corrected) - ...
        (q3 * gyro_y_corrected);
    q2 = q2 + (qa * gyro_y_corrected) - (qb * gyro_z_corrected) + ...
        (q3 * gyro_x_corrected);
    q3 = q3 + (qa * gyro_z_corrected) + (qb * gyro_y_corrected) - ...
        (qc * gyro_x_corrected);
    
    %Normalize quaternion
    quaternion_mag = ( (q0 * q0) + (q1 * q1) + (q2 * q2) + (q3 * q3) ) ^ 0.5;
    q0 = q0 / quaternion_mag;
    q1 = q1 / quaternion_mag;
    q2 = q2 / quaternion_mag;
    q3 = q3 / quaternion_mag;
    
    %Estimate the gravity direction from the quaternion values
    grav_x = 2 * ( (q1 * q3) - (q0 * q2) );
    grav_y = 2 * ( (q0 * q1) + (q2 * q3) );
    grav_z = (q0 * q0) - (q1 * q1) - (q2 * q2) + (q3 * q3);
    
    %Limit the gravity vector in x-direction to maintain a magnitude of 1
%     grav_x = min( grav_x , 1 );
%     grav_x = max( grav_x , -1 );

    %Normalize the gravity vector
    grav_mag = sqrt( ( grav_x * grav_x ) + ( grav_y * grav_y ) + ...
        ( grav_z * grav_z ) );
    grav_x = grav_x / grav_mag;
    grav_y = grav_y / grav_mag;
    grav_z = grav_z / grav_mag;
    
    %Calculate the pitch, roll, and yaw
    yaw = atan2( 2 * ( (q0 * q3) + (q1 * q2) ) , ...
        (q0 * q0) + (q1 * q1) - (q2 * q2) - (q3 * q3) );
    pitch = asin( (-1) * grav_x );
    roll = atan2( grav_y , grav_z );
    
    %Create a vector of current integral feedback terms to output
    integralFeedback = [ integralFeedback_x ; ...
        integralFeedback_y ; integralFeedback_z ];
    
    %Create a vector of the corrected gyroscope terms
    %gyroReadings_corrected = [ gyro_x_corrected ; ...
    %    gyro_y_corrected ; gyro_z_corrected ];
    
    %Create a vector of the newly calculated quaternion values
    quaternions = [ q0 ; q1 ; q2 ; q3 ];
    
    %Create a vector of the calculated Euler angles
    eulerAngles = [ roll ;  pitch ; yaw ];
    
end %function
